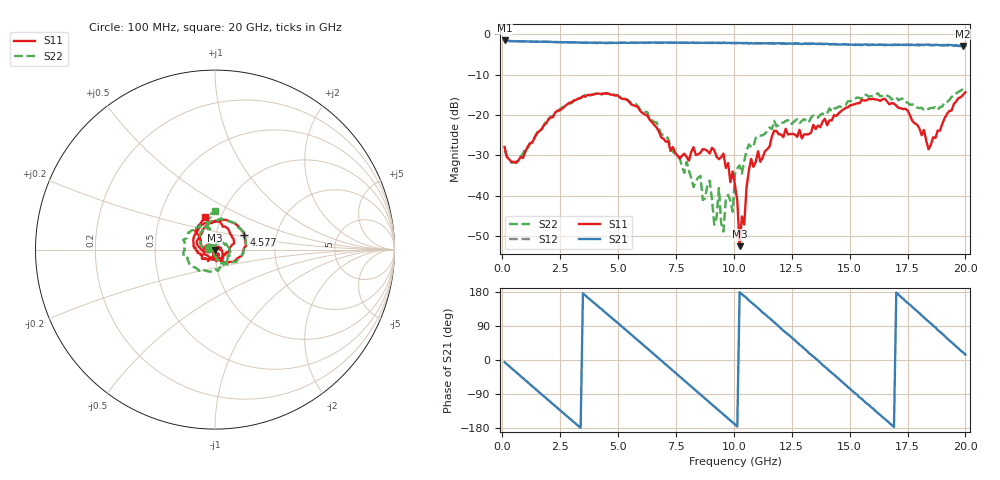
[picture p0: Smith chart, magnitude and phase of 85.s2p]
!Agilent Technologies,N5230C,MY49001569,A.09.33.09
!Agilent N5230C: A.09.33.09
!Date: Monday, July 27, 2015 14:15:37
!Correction: S11(Full 2 Port(1,2))
!S21(Full 2 Port(1,2))
!S12(Full 2 Port(1,2))
!S22(Full 2 Port(1,2))
!S2P File: Measurements: S11, S21, S12, S22:
# Hz S  dB  R 50
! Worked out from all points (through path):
!   201 points, 100 MHz to 20 GHz, reference 50 ohm
!   highest |S21| = -1.56 dB at 100 MHz (marker M1); lowest = -3.0 dB at 19.9 GHz (marker M2)
!   group delay of S21, straight-line fit = 148 ps
!   lowest |S11| = -52.5 dB at 10.25 GHz (marker M3), VSWR 1.00, Z = 49.8 - j0.155 ohm
!   |S11| at or under -10 dB: start of sweep to end of sweep
!   |S22| runs from -48.9 to -13.4 dB; largest |S21 - S12| = 0.025
!   S11 on the Smith chart (normalised r, x): 100 MHz: 0.92, +0.01; 4.577 GHz: 1.37, +0.23; 20 GHz: 0.84, +0.32
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1e8  -27.97 169.0  -1.56 -5.8  -1.58 -5.6  -28.91 165.2
1.692e9  -23.59 170.2  -1.87 -90.2  -1.90 -90.4  -23.65 170.9
3.483e9  -15.34 81.0  -2.13 175.8  -2.13 175.5  -15.52 83.9
4.5775e9  -14.73 26.6  -2.21 118.7  -2.14 119.0  -14.79 29.5
6.7665e9  -24.19 -65.7  -2.11 3.8  -2.11 3.8  -23.42 -69.1
8.259e9  -28.00 -64.2  -2.11 -75.3  -2.12 -75.3  -37.89 -103.4
8.9555e9  -29.57 -70.7  -2.16 -112.2  -2.17 -111.9  -36.30 -95.3
9.1545e9  -28.73 -92.0  -2.14 -122.7  -2.12 -122.7  -47.20 -128.1
9.3535e9  -30.99 -88.5  -2.13 -133.2  -2.20 -133.4  -38.14 -133.2
9.5525e9  -29.57 -107.0  -2.09 -144.0  -2.17 -143.8  -48.91 124.3
9.652e9  -33.16 -115.2  -2.20 -149.4  -2.20 -148.9  -40.92 133.4
9.9505e9  -34.02 -113.7  -2.17 -164.8  -2.20 -164.9  -44.01 110.5
1.005e10  -37.46 -132.8  -2.19 -170.4  -2.24 -169.9  -34.59 95.0
1.0249e10  -52.53 -138.7  -2.19 179.1  -2.22 179.5  -32.50 108.5
1.07465e10  -30.92 32.9  -2.21 152.6  -2.26 152.6  -27.99 65.9
1.21395e10  -25.54 -33.3  -2.37 77.5  -2.24 78.5  -21.97 3.0
1.3433e10  -22.46 -121.3  -2.31 9.2  -2.42 9.3  -20.16 -50.6
1.51245e10  -17.51 153.7  -2.61 -82.1  -2.40 -81.2  -16.41 -139.4
1.67165e10  -17.38 71.4  -2.66 -166.3  -2.65 -166.3  -15.47 140.1
1.8408e10  -28.51 -76.9  -2.65 101.3  -2.60 102.2  -18.49 106.2
1.99005e10  -15.01 112.6  -2.96 20.2  -3.11 20.4  -13.51 90.3
2e10  -14.37 107.3  -2.93 14.2  -2.92 14.0  -13.41 89.4
